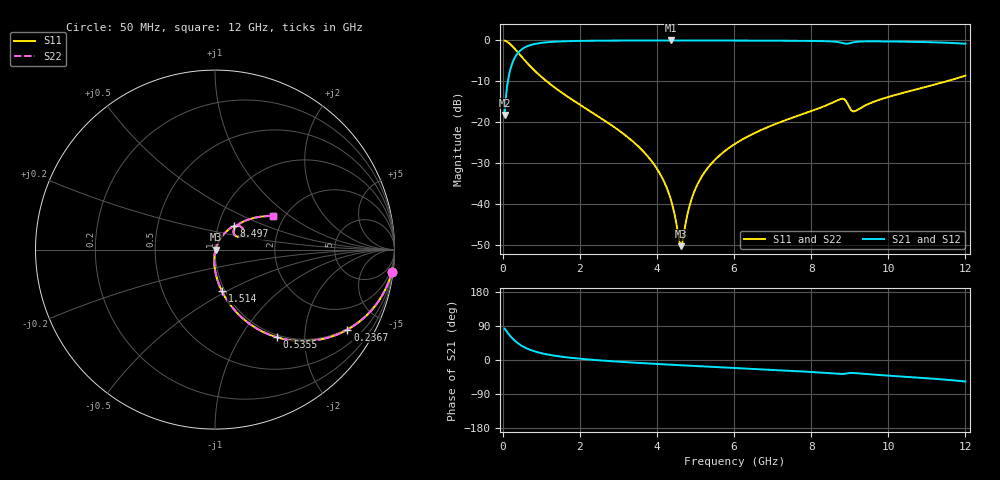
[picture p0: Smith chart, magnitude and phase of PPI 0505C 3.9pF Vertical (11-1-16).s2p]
# GHz S MA R 50
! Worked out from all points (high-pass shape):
!   1601 points, 50 MHz to 12 GHz, reference 50 ohm
!   highest |S21| = -0.03 dB at 4.374 GHz (marker M1); lowest = -18.2 dB at 50 MHz (marker M2)
!   |S21| within 3 dB of the highest: 400.2 MHz to end of sweep
!   lowest |S11| = -50.2 dB at 4.621 GHz (marker M3), VSWR 1.01, Z = 50.3 - j0.0862 ohm
!   |S11| at or under -10 dB: 1.143 GHz to 11.51 GHz (10.36 GHz wide, 164 % of centre)
!   |S22| runs from -50.2 to -0.1 dB; largest |S21 - S12| = 0
!   S11 on the Smith chart (normalised r, x): 50 MHz: 1, -16; 236.7 MHz: 0.96, -3.34; 535.5 MHz: 0.96, -1.46; 1.514 GHz: 0.97, -0.47; 8.497 GHz: 1.19, +0.32; 12 GHz: 1.74, +0.75
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0.05  0.9924 -7.2  0.1228 82.8  0.1228 82.8  0.9924 -7.2
0.1470937  0.9395 -20.5  0.3422 69.5  0.3422 69.5  0.9395 -20.5
0.2367188  0.8622 -31.1  0.5061 58.8  0.5061 58.8  0.8622 -31.1
0.5354688  0.5973 -54.8  0.801 35.1  0.801 35.1  0.5973 -54.8
0.9089063  0.3938 -69.4  0.9178 20.4  0.9178 20.4  0.3938 -69.4
1.513875  0.2336 -80.6  0.9704 8.9  0.9704 8.9  0.2336 -80.6
2.044156  0.1595 -86.2  0.985 3.0  0.985 3.0  0.1595 -86.2
3.33625  0.06066 -94.1  0.9953 -6.6  0.9953 -6.6  0.06066 -94.1
4.038312  0.02552 -94.2  0.9965 -10.7  0.9965 -10.7  0.02552 -94.2
4.374406  0.01091 -86.6  0.9967 -12.5  0.9967 -12.5  0.01091 -86.6
4.620875  0.003096 -16.1  0.9966 -13.9  0.9966 -13.9  0.003096 -16.1
4.673156  0.003719 19.0  0.9966 -14.1  0.9966 -14.1  0.003719 19.0
4.874812  0.01069 57.4  0.9964 -15.2  0.9964 -15.2  0.01069 57.4
5.106344  0.01965 64.0  0.9962 -16.4  0.9962 -16.4  0.01965 64.0
5.48725  0.03429 65.8  0.9956 -18.4  0.9956 -18.4  0.03429 65.8
6.025  0.05471 65.0  0.9944 -21.1  0.9944 -21.1  0.05471 65.0
8.019156  0.1383 55.6  0.9834 -31.8  0.9834 -31.8  0.1383 55.6
8.497156  0.1693 50.5  0.9717 -34.9  0.9717 -34.9  0.1693 50.5
8.825781  0.1939 36.4  0.9261 -36.8  0.9261 -36.8  0.1939 36.4
9.124531  0.1366 38.8  0.9515 -34.5  0.9515 -34.5  0.1366 38.8
10.01331  0.2048 46.2  0.9692 -41.3  0.9692 -41.3  0.2048 46.2
12  0.3712 30.2  0.9089 -56.8  0.9089 -56.8  0.3712 30.2
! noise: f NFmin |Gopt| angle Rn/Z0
0.05  0.0005929  0.9202  1.991  0.001643
1.372  0.004956  0.7297  4.92  0.003644
2.701  0.008067  0.6822  8.571  0.004889
4.031  0.01089  0.6552  12.25  0.00595
5.36  0.01367  0.6398  15.88  0.007032
6.682  0.01675  0.6364  19.45  0.008441
8.012  0.02286  0.6753  23.16  0.01305
9.341  0.04082  0.7767  27.3  0.03535
10.67  0.03171  0.6906  30.31  0.01863
12  0.04903  0.767  34.21  0.03918
